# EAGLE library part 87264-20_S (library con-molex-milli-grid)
RECEPTACAL
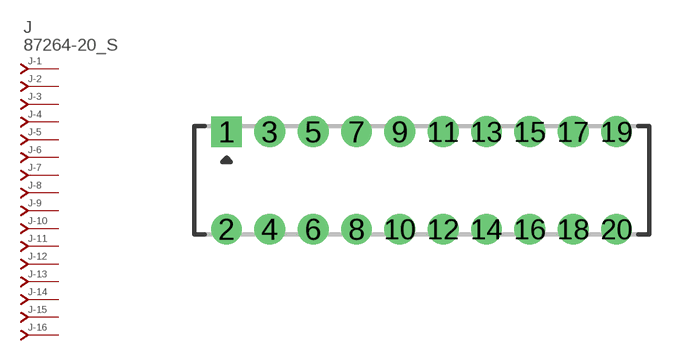
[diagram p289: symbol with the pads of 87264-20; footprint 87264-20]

Designator prefix J; gates -1=J-NV -2=J-N -3=J-N -4=J-N -5=J-N -6=J-N -7=J-N -8=J-N -9=J-N -10=J-N -11=J-N -12=J-N -13=J-N -14=J-N -15=J-N -16=J-N -17=J-N -18=J-N -19=J-N -20=J-N

## 87264-20_S  [87264-20]
1  -1:J  pas
2  -2:J  pas
3  -3:J  pas
4  -4:J  pas
5  -5:J  pas
6  -6:J  pas
7  -7:J  pas
8  -8:J  pas
9  -9:J  pas
10  -10:J  pas
11  -11:J  pas
12  -12:J  pas
13  -13:J  pas
14  -14:J  pas
15  -15:J  pas
16  -16:J  pas
17  -17:J  pas
18  -18:J  pas
19  -19:J  pas
20  -20:J  pas

## Footprint 87264-20 (pad centres in mm)
RECEPTACAL Dual Row, Side Entry
drill 0.914 square: 1 -9,2.25
drill 0.914: 2 -9,-2.25; 3 -7,2.25; 4 -7,-2.25; 5 -5,2.25; 6 -5,-2.25; 7 -3,2.25; 8 -3,-2.25; 9 -1,2.25; 10 -1,-2.25; 11 1,2.25; 12 1,-2.25; 13 3,2.25; 14 3,-2.25; 15 5,2.25; 16 5,-2.25; 17 7,2.25; 18 7,-2.25; 19 9,2.25; 20 9,-2.25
